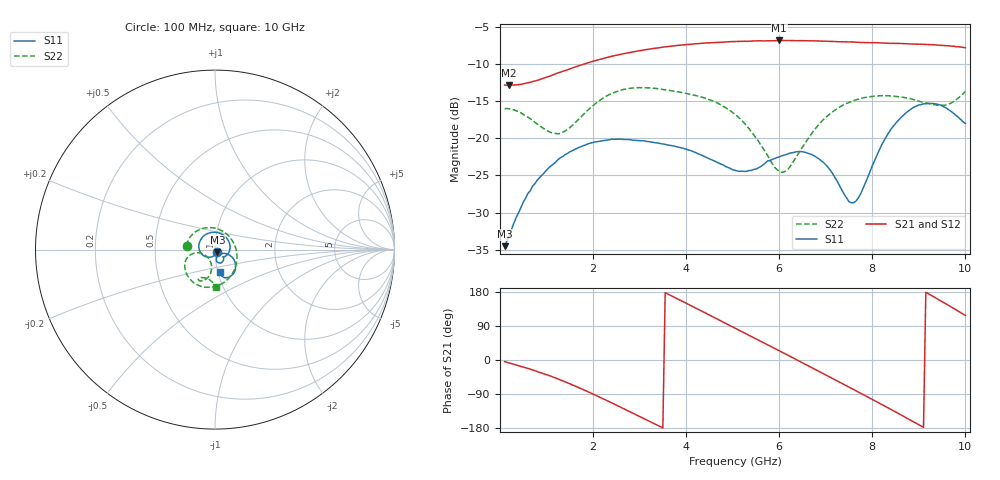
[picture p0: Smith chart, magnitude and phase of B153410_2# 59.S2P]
!  2-Port S-parameters saved by WinCal
! VAR MeasName=S-Parameters (CALIBRATED_DATA) read from VNA (N5245A)
! VAR MeasDate=2016-12-23 10:02:31
! VAR NAME=B153410_2# 59
! VAR FILENAME=B153410_2# 59.S2P
! VAR DATE=2016-12-23 10:02:31
! VAR PHYS_PORTS=1,2
# Hz S DB R 50
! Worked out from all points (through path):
!   199 points, 100 MHz to 10 GHz, reference 50 ohm
!   highest |S21| = -6.80 dB at 6 GHz (marker M1); lowest = -12.8 dB at 200 MHz (marker M2)
!   group delay of S21, straight-line fit = 171 ps
!   lowest |S11| = -34.5 dB at 100 MHz (marker M3), VSWR 1.04, Z = 51.4 - j1.31 ohm
!   |S11| at or under -10 dB: start of sweep to end of sweep
!   |S22| runs from -24.6 to -13.2 dB; largest |S21 - S12| = 0.0031
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1e8  -34.53 -43.0  -12.82 -4.2  -12.84 -4.3  -15.99 172.2
2e8  -33.19 -64.4  -12.85 -7.8  -12.83 -7.9  -16.02 163.2
5e8  -28.62 -103.1  -12.65 -18.5  -12.65 -18.5  -16.77 134.5
8e8  -25.64 -125.2  -12.19 -30.0  -12.20 -30.0  -18.07 101.4
1.25e9  -22.85 -151.3  -11.18 -50.2  -11.18 -50.2  -19.38 36.2
1.75e9  -21.09 178.5  -10.10 -75.9  -10.11 -76.0  -17.07 -31.5
2.55e9  -20.11 124.0  -8.72 -121.8  -8.75 -121.9  -13.59 -94.1
3.4e9  -20.63 55.0  -7.81 -173.1  -7.81 -173.0  -13.33 -130.2
4.15e9  -21.79 -4.4  -7.27 140.5  -7.27 140.6  -14.15 -148.8
4.6e9  -23.03 -29.5  -7.09 112.5  -7.09 112.6  -15.03 -158.7
5.05e9  -24.30 -41.8  -6.95 84.3  -6.96 84.5  -16.75 -167.4
5.5e9  -24.15 -42.8  -6.87 56.1  -6.86 56.2  -19.94 -169.9
6e9  -22.51 -51.5  -6.80 24.6  -6.81 24.7  -24.45 -142.7
6.2e9  -22.07 -56.8  -6.81 11.7  -6.82 11.8  -24.08 -121.9
6.7e9  -22.19 -73.6  -6.85 -20.2  -6.86 -20.1  -19.32 -99.9
7.2e9  -25.31 -82.3  -6.94 -52.3  -6.95 -52.2  -16.17 -103.3
7.6e9  -28.67 -52.7  -7.01 -78.0  -7.04 -77.9  -14.90 -109.2
8.35e9  -19.27 -25.2  -7.18 -127.1  -7.17 -126.8  -14.25 -117.6
8.75e9  -16.43 -40.6  -7.24 -153.9  -7.25 -153.6  -14.56 -119.2
9.2e9  -15.29 -59.9  -7.36 175.3  -7.35 175.4  -15.29 -115.2
9.65e9  -16.19 -75.0  -7.53 143.2  -7.53 143.4  -15.37 -100.5
1e10  -18.00 -76.2  -7.79 117.4  -7.79 117.6  -13.67 -87.7
